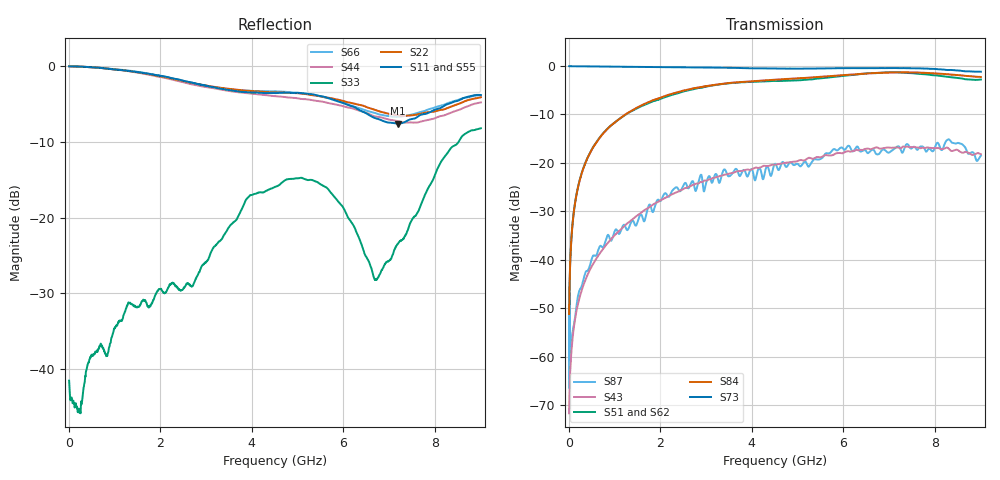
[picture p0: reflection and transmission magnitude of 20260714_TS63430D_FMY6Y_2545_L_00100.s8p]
# GHz S DB R 50
! CMT, SN0916, 25263762, 26.7.0
! Date: 15.07.2026 14:53:44
! Data: Format
! Freq S1.1:dB/Ang S1.2:dB/Ang S1.3:dB/Ang S1.4:dB/Ang S1.5:dB/Ang S1.6:dB/Ang S1.7:dB/Ang S1.8:dB/Ang
!  S2.1:dB/Ang S2.2:dB/Ang S2.3:dB/Ang S2.4:dB/Ang S2.5:dB/Ang S2.6:dB/Ang S2.7:dB/Ang S2.8:dB/Ang
!  S3.1:dB/Ang S3.2:dB/Ang S3.3:dB/Ang S3.4:dB/Ang S3.5:dB/Ang S3.6:dB/Ang S3.7:dB/Ang S3.8:dB/Ang
!  S4.1:dB/Ang S4.2:dB/Ang S4.3:dB/Ang S4.4:dB/Ang S4.5:dB/Ang S4.6:dB/Ang S4.7:dB/Ang S4.8:dB/Ang
!  S5.1:dB/Ang S5.2:dB/Ang S5.3:dB/Ang S5.4:dB/Ang S5.5:dB/Ang S5.6:dB/Ang S5.7:dB/Ang S5.8:dB/Ang
!  S6.1:dB/Ang S6.2:dB/Ang S6.3:dB/Ang S6.4:dB/Ang S6.5:dB/Ang S6.6:dB/Ang S6.7:dB/Ang S6.8:dB/Ang
!  S7.1:dB/Ang S7.2:dB/Ang S7.3:dB/Ang S7.4:dB/Ang S7.5:dB/Ang S7.6:dB/Ang S7.7:dB/Ang S7.8:dB/Ang
!  S8.1:dB/Ang S8.2:dB/Ang S8.3:dB/Ang S8.4:dB/Ang S8.5:dB/Ang S8.6:dB/Ang S8.7:dB/Ang S8.8:dB/Ang
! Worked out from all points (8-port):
!   2001 points, 10 MHz to 9 GHz, reference 50 ohm
!   strongest paths, dB at 10 MHz, 2.257 GHz, 4.505 GHz, 6.753 GHz, 9 GHz:
!     S73: -0.1, -0.3, -0.5, -0.5, -1.2
!     S84: -51.2, -5.8, -2.9, -1.4, -2.3
!     S51: -50.8, -6.0, -3.1, -1.5, -2.8
!     S62: -51.0, -5.9, -3.3, -1.8, -2.7
!     S43: -71.6, -26.5, -20.4, -16.9, -18.2
!     S87: -51.9, -25.8, -20.2, -18.2, -18.5
!   lowest |S11| = -7.6 dB at 7.184 GHz (marker M1), VSWR 2.43, Z = 21.4 - j9.38 ohm
!   |S11| at or under -10 dB: nowhere
